PROGRAM P_Prog6
VAR

	fbKL6401 					: FB_LON_KL6401;

	fbREAD_159		: FB_READ_159_SNVT_pump_sensor;
	fbSEND_159		: FB_SEND_159_SNVT_pump_sensor;

	fbREAD_160		: FB_READ_160_SNVT_abs_humid;
	fbSEND_160		: FB_SEND_160_SNVT_abs_humid;

	fbREAD_161		: FB_READ_161_SNVT_flow_p;
	fbSEND_161		: FB_SEND_161_SNVT_flow_p;

	fbREAD_162		: FB_READ_162_SNVT_dev_c_mode;
	fbSEND_162		: FB_SEND_162_SNVT_dev_c_mode;

	fbREAD_163		: FB_READ_163_SNVT_valve_mode;
	fbSEND_163		: FB_SEND_163_SNVT_valve_mode;

	fbREAD_164		: FB_READ_164_SNVT_alarm_2;
	fbSEND_164		: FB_SEND_164_SNVT_alarm_2;

	fbREAD_165		: FB_READ_165_SNVT_state_64;
	fbSEND_165		: FB_SEND_165_SNVT_state_64;

	fbREAD_166		: FB_READ_166_SNVT_nv_type;
	fbSEND_166		: FB_SEND_166_SNVT_nv_type;
(*
	fbREAD_167		: FB_READ_109_SNVT_occupancy;
	fbSEND_167		: FB_SEND_109_SNVT_occupancy;
*)
	fbREAD_168		: FB_READ_168_SNVT_ent_opmode;
	fbSEND_168		: FB_SEND_168_SNVT_ent_opmode;

	fbREAD_169		: FB_READ_169_SNVT_ent_state;
	fbSEND_169		: FB_SEND_169_SNVT_ent_state;

	fbREAD_170		: FB_READ_170_SNVT_ent_status;
	fbSEND_170		: FB_SEND_170_SNVT_ent_status;

	fbREAD_171		: FB_READ_171_SNVT_flow_dir;
	fbSEND_171		: FB_SEND_171_SNVT_flow_dir;

	fbREAD_172		: FB_READ_172_SNVT_hvac_satsts;
	fbSEND_172		: FB_SEND_172_SNVT_hvac_satsts;

	fbREAD_173		: FB_READ_173_SNVT_dev_status;
	fbSEND_173		: FB_SEND_173_SNVT_dev_status;

	fbREAD_174		: FB_READ_174_SNVT_dev_fault;
	fbSEND_174		: FB_SEND_174_SNVT_dev_fault;

	fbREAD_175		: FB_READ_175_SNVT_dev_maint;
	fbSEND_175		: FB_SEND_175_SNVT_dev_maint;

	fbREAD_176		: FB_READ_176_SNVT_date_event;
	fbSEND_176		: FB_SEND_176_SNVT_date_event;

	fbREAD_177		: FB_READ_177_SNVT_sched_val;
	fbSEND_177		: FB_SEND_177_SNVT_sched_val;

(*
	fbREAD_178		: FB_READ_178;
	fbSEND_178		: FB_SEND_146_SNVT_elec_kwh_l;

	fbREAD_179		: FB_READ_147_SNVT_temp_diff_p;
	fbSEND_179		: FB_SEND_147_SNVT_temp_diff_p;
*)
	fbREAD_180		: FB_READ_180_SNVT_sblnd_state;
	fbSEND_180		: FB_SEND_180_SNVT_sblnd_state;

	fbREAD_181		: FB_READ_181_SNVT_rac_ctrl;
	fbSEND_181		: FB_SEND_181_SNVT_rac_ctrl;

	fbREAD_182		: FB_READ_182_SNVT_rac_req;
	fbSEND_182		: FB_SEND_182_SNVT_rac_req;

	fbREAD_183		: FB_READ_183_SNVT_count_32;
	fbSEND_183		: FB_SEND_183_SNVT_count_32;

	fbREAD_184		: FB_READ_184_SNVT_clothes_w_c;
	fbSEND_184		: FB_SEND_184_SNVT_clothes_w_c;

	fbREAD_185		: FB_READ_185_SNVT_clothes_w_m;
	fbSEND_185		: FB_SEND_185_SNVT_clothes_w_m;

	fbREAD_186		: FB_READ_186_SNVT_clothes_w_s;
	fbSEND_186		: FB_SEND_186_SNVT_clothes_w_s;

	fbREAD_187		: FB_READ_187_SNVT_clothes_w_a;
	fbSEND_187		: FB_SEND_187_SNVT_clothes_w_a;

	fbREAD_188		: FB_READ_188_SNVT_multiplier_s;
	fbSEND_188		: FB_SEND_188_SNVT_multiplier_s;

	fbREAD_189		: FB_READ_189_SNVT_switch_2;
	fbSEND_189		: FB_SEND_189_SNVT_switch_2;

	fbREAD_190		: FB_READ_190_SNVT_color_2;
	fbSEND_190		: FB_SEND_190_SNVT_color_2;

END_VAR

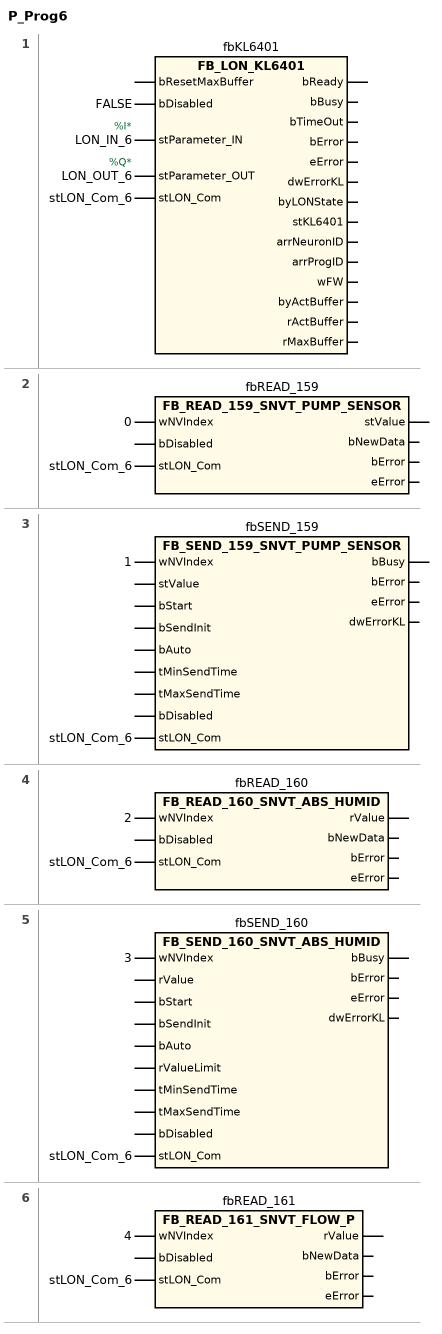
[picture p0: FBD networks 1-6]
// NETWORK 1
//   LON_IN_6: AT %I*
//   LON_OUT_6: AT %Q*
fbKL6401(
    bDisabled := FALSE,
    stParameter_IN := LON_IN_6,
    stParameter_OUT := LON_OUT_6,
    stLON_Com := stLON_Com_6); // FB_LON_KL6401

// NETWORK 2
fbREAD_159(wNVIndex := 0, stLON_Com := stLON_Com_6); // FB_READ_159_SNVT_PUMP_SENSOR

// NETWORK 3
fbSEND_159(wNVIndex := 1, stLON_Com := stLON_Com_6); // FB_SEND_159_SNVT_PUMP_SENSOR

// NETWORK 4
fbREAD_160(wNVIndex := 2, stLON_Com := stLON_Com_6); // FB_READ_160_SNVT_ABS_HUMID

// NETWORK 5
fbSEND_160(wNVIndex := 3, stLON_Com := stLON_Com_6); // FB_SEND_160_SNVT_ABS_HUMID

// NETWORK 6
fbREAD_161(wNVIndex := 4, stLON_Com := stLON_Com_6); // FB_READ_161_SNVT_FLOW_P

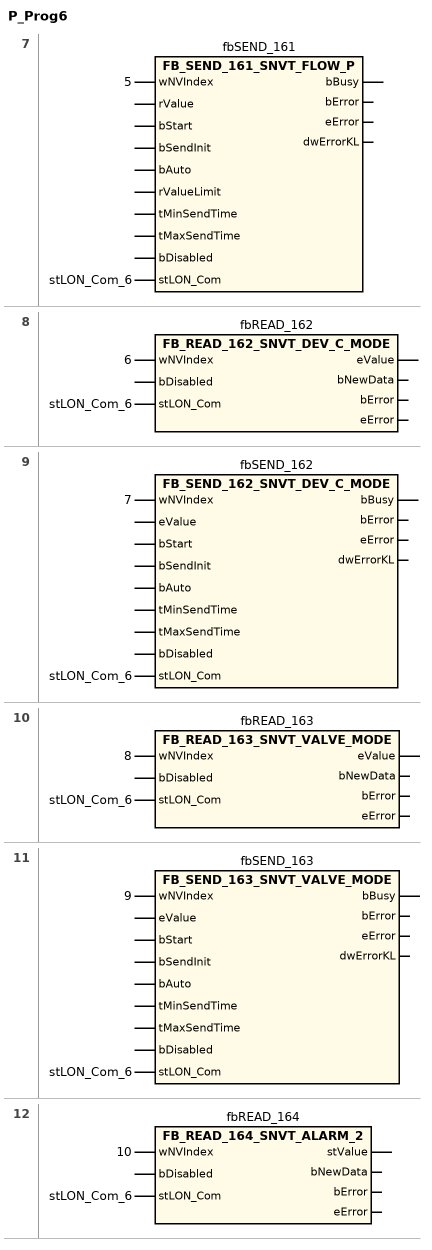
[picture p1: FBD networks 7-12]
// NETWORK 7
fbSEND_161(wNVIndex := 5, stLON_Com := stLON_Com_6); // FB_SEND_161_SNVT_FLOW_P

// NETWORK 8
fbREAD_162(wNVIndex := 6, stLON_Com := stLON_Com_6); // FB_READ_162_SNVT_DEV_C_MODE

// NETWORK 9
fbSEND_162(wNVIndex := 7, stLON_Com := stLON_Com_6); // FB_SEND_162_SNVT_DEV_C_MODE

// NETWORK 10
fbREAD_163(wNVIndex := 8, stLON_Com := stLON_Com_6); // FB_READ_163_SNVT_VALVE_MODE

// NETWORK 11
fbSEND_163(wNVIndex := 9, stLON_Com := stLON_Com_6); // FB_SEND_163_SNVT_VALVE_MODE

// NETWORK 12
fbREAD_164(wNVIndex := 10, stLON_Com := stLON_Com_6); // FB_READ_164_SNVT_ALARM_2

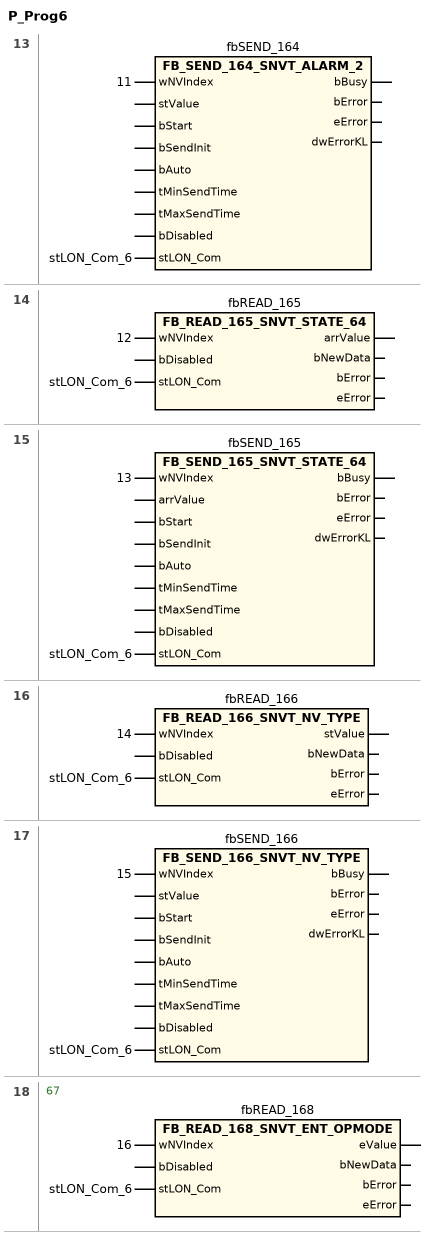
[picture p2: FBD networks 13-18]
// NETWORK 13
fbSEND_164(wNVIndex := 11, stLON_Com := stLON_Com_6); // FB_SEND_164_SNVT_ALARM_2

// NETWORK 14
fbREAD_165(wNVIndex := 12, stLON_Com := stLON_Com_6); // FB_READ_165_SNVT_STATE_64

// NETWORK 15
fbSEND_165(wNVIndex := 13, stLON_Com := stLON_Com_6); // FB_SEND_165_SNVT_STATE_64

// NETWORK 16
fbREAD_166(wNVIndex := 14, stLON_Com := stLON_Com_6); // FB_READ_166_SNVT_NV_TYPE

// NETWORK 17
fbSEND_166(wNVIndex := 15, stLON_Com := stLON_Com_6); // FB_SEND_166_SNVT_NV_TYPE

// NETWORK 18
// 					67
//
//
//   fbREAD_168: fbREAD_167 : FB_READ_109_SNVT_occupancy; fbSEND_167 : FB_SEND_109_SNVT_occupancy;
fbREAD_168(wNVIndex := 16, stLON_Com := stLON_Com_6); // FB_READ_168_SNVT_ENT_OPMODE

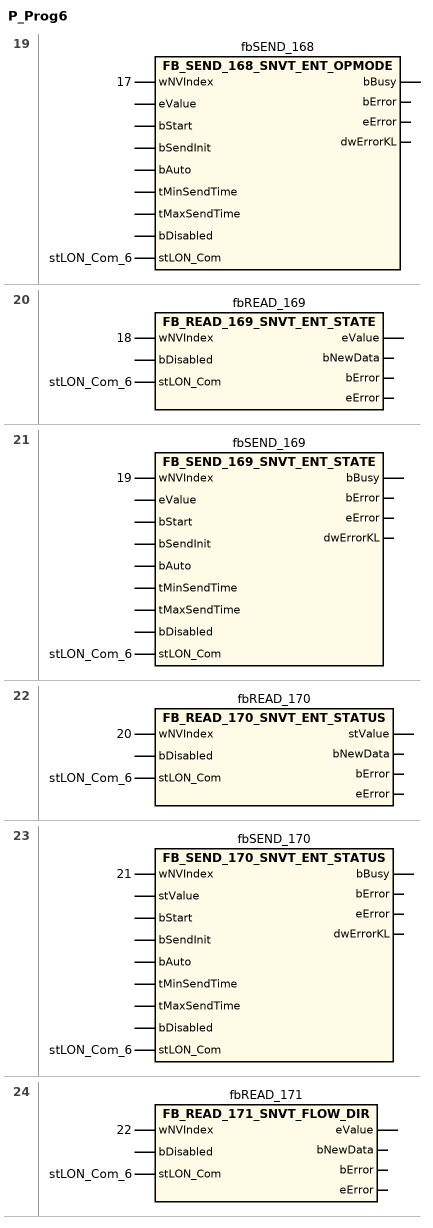
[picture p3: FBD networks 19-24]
// NETWORK 19
fbSEND_168(wNVIndex := 17, stLON_Com := stLON_Com_6); // FB_SEND_168_SNVT_ENT_OPMODE

// NETWORK 20
fbREAD_169(wNVIndex := 18, stLON_Com := stLON_Com_6); // FB_READ_169_SNVT_ENT_STATE

// NETWORK 21
fbSEND_169(wNVIndex := 19, stLON_Com := stLON_Com_6); // FB_SEND_169_SNVT_ENT_STATE

// NETWORK 22
fbREAD_170(wNVIndex := 20, stLON_Com := stLON_Com_6); // FB_READ_170_SNVT_ENT_STATUS

// NETWORK 23
fbSEND_170(wNVIndex := 21, stLON_Com := stLON_Com_6); // FB_SEND_170_SNVT_ENT_STATUS

// NETWORK 24
fbREAD_171(wNVIndex := 22, stLON_Com := stLON_Com_6); // FB_READ_171_SNVT_FLOW_DIR

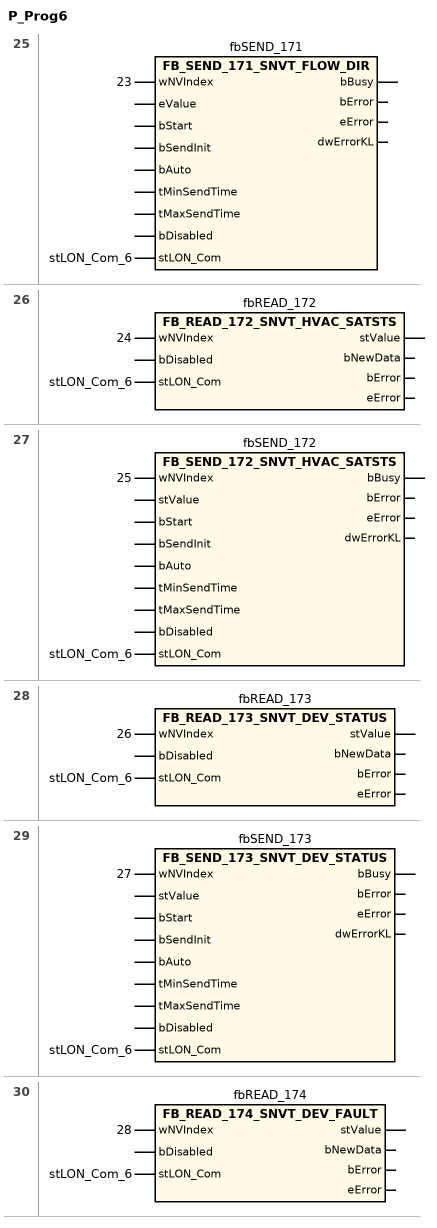
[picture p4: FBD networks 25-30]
// NETWORK 25
fbSEND_171(wNVIndex := 23, stLON_Com := stLON_Com_6); // FB_SEND_171_SNVT_FLOW_DIR

// NETWORK 26
fbREAD_172(wNVIndex := 24, stLON_Com := stLON_Com_6); // FB_READ_172_SNVT_HVAC_SATSTS

// NETWORK 27
fbSEND_172(wNVIndex := 25, stLON_Com := stLON_Com_6); // FB_SEND_172_SNVT_HVAC_SATSTS

// NETWORK 28
fbREAD_173(wNVIndex := 26, stLON_Com := stLON_Com_6); // FB_READ_173_SNVT_DEV_STATUS

// NETWORK 29
fbSEND_173(wNVIndex := 27, stLON_Com := stLON_Com_6); // FB_SEND_173_SNVT_DEV_STATUS

// NETWORK 30
fbREAD_174(wNVIndex := 28, stLON_Com := stLON_Com_6); // FB_READ_174_SNVT_DEV_FAULT

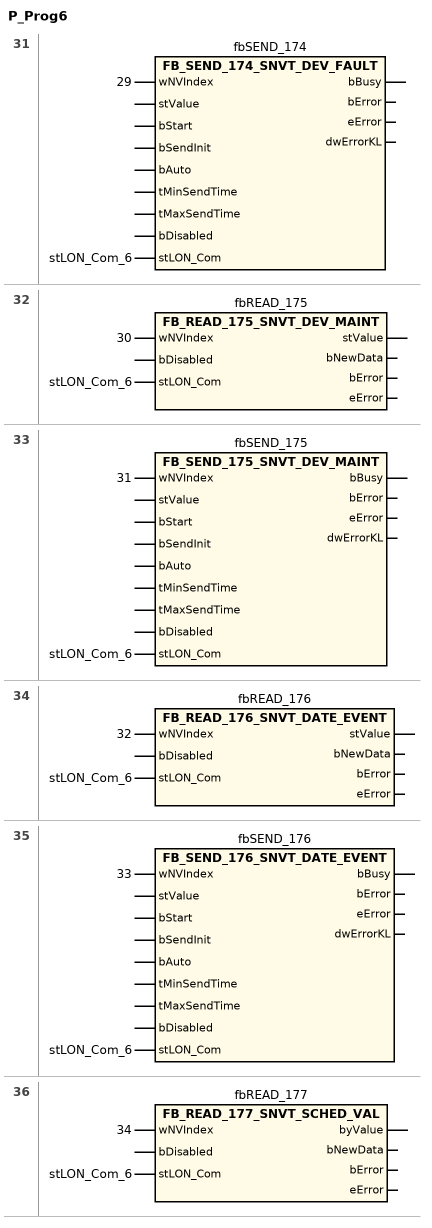
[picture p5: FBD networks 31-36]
// NETWORK 31
fbSEND_174(wNVIndex := 29, stLON_Com := stLON_Com_6); // FB_SEND_174_SNVT_DEV_FAULT

// NETWORK 32
fbREAD_175(wNVIndex := 30, stLON_Com := stLON_Com_6); // FB_READ_175_SNVT_DEV_MAINT

// NETWORK 33
fbSEND_175(wNVIndex := 31, stLON_Com := stLON_Com_6); // FB_SEND_175_SNVT_DEV_MAINT

// NETWORK 34
fbREAD_176(wNVIndex := 32, stLON_Com := stLON_Com_6); // FB_READ_176_SNVT_DATE_EVENT

// NETWORK 35
fbSEND_176(wNVIndex := 33, stLON_Com := stLON_Com_6); // FB_SEND_176_SNVT_DATE_EVENT

// NETWORK 36
fbREAD_177(wNVIndex := 34, stLON_Com := stLON_Com_6); // FB_READ_177_SNVT_SCHED_VAL

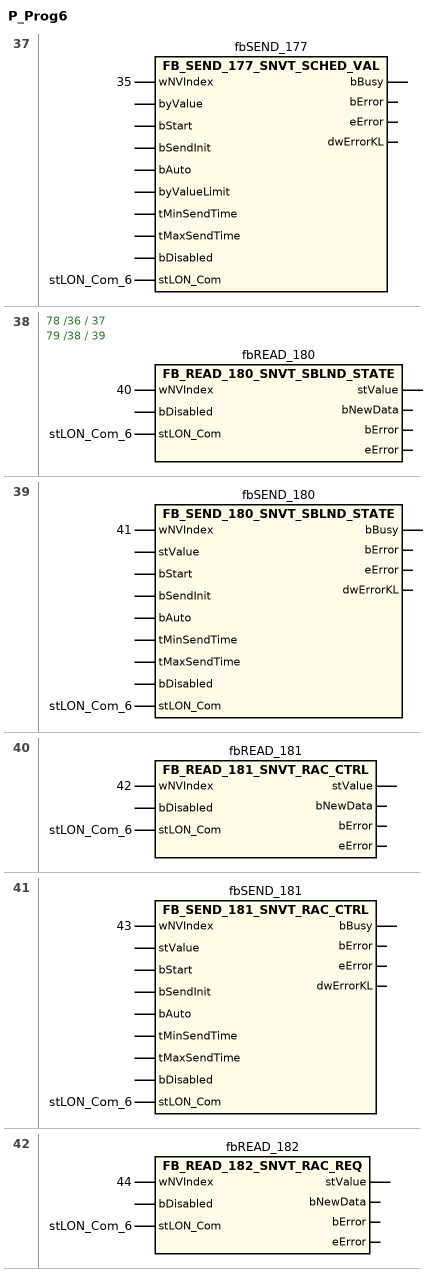
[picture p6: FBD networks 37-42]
// NETWORK 37
fbSEND_177(wNVIndex := 35, stLON_Com := stLON_Com_6); // FB_SEND_177_SNVT_SCHED_VAL

// NETWORK 38
// 					78 /36 / 37
// 79 /38 / 39
//
//
//   fbREAD_180: fbREAD_178 : FB_READ_178; fbSEND_178 : FB_SEND_146_SNVT_elec_kwh_l; fbREAD_179 : FB_READ_147_SNVT_temp_diff_p; fbSEND_179 : FB_SEND_147_SNVT_temp_diff_p;
fbREAD_180(wNVIndex := 40, stLON_Com := stLON_Com_6); // FB_READ_180_SNVT_SBLND_STATE

// NETWORK 39
fbSEND_180(wNVIndex := 41, stLON_Com := stLON_Com_6); // FB_SEND_180_SNVT_SBLND_STATE

// NETWORK 40
fbREAD_181(wNVIndex := 42, stLON_Com := stLON_Com_6); // FB_READ_181_SNVT_RAC_CTRL

// NETWORK 41
fbSEND_181(wNVIndex := 43, stLON_Com := stLON_Com_6); // FB_SEND_181_SNVT_RAC_CTRL

// NETWORK 42
fbREAD_182(wNVIndex := 44, stLON_Com := stLON_Com_6); // FB_READ_182_SNVT_RAC_REQ

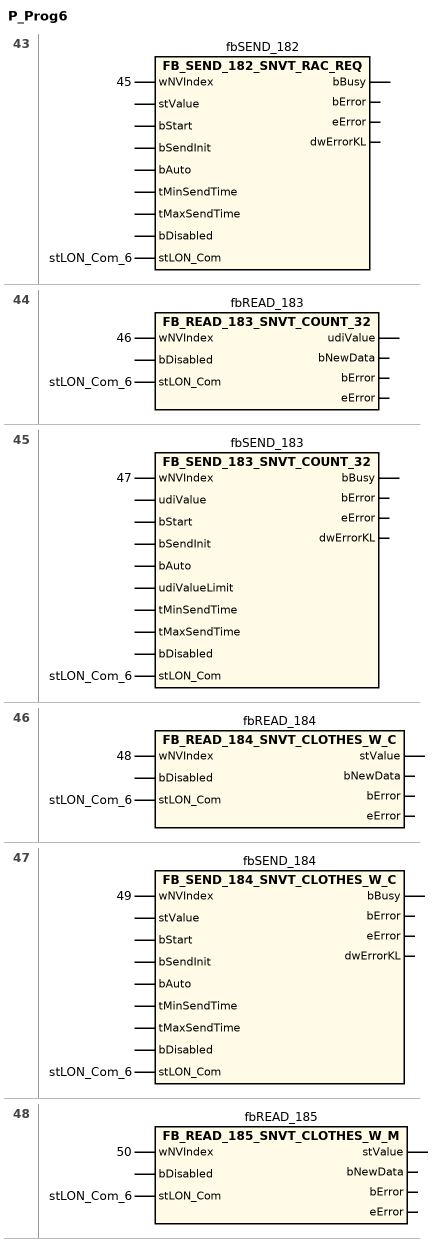
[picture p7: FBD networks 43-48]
// NETWORK 43
fbSEND_182(wNVIndex := 45, stLON_Com := stLON_Com_6); // FB_SEND_182_SNVT_RAC_REQ

// NETWORK 44
fbREAD_183(wNVIndex := 46, stLON_Com := stLON_Com_6); // FB_READ_183_SNVT_COUNT_32

// NETWORK 45
fbSEND_183(wNVIndex := 47, stLON_Com := stLON_Com_6); // FB_SEND_183_SNVT_COUNT_32

// NETWORK 46
fbREAD_184(wNVIndex := 48, stLON_Com := stLON_Com_6); // FB_READ_184_SNVT_CLOTHES_W_C

// NETWORK 47
fbSEND_184(wNVIndex := 49, stLON_Com := stLON_Com_6); // FB_SEND_184_SNVT_CLOTHES_W_C

// NETWORK 48
fbREAD_185(wNVIndex := 50, stLON_Com := stLON_Com_6); // FB_READ_185_SNVT_CLOTHES_W_M

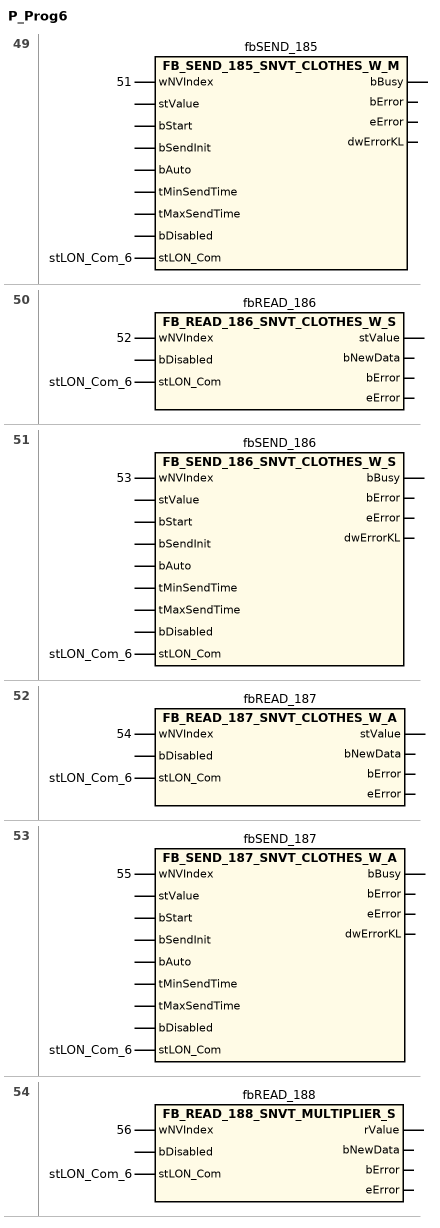
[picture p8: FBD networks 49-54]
// NETWORK 49
fbSEND_185(wNVIndex := 51, stLON_Com := stLON_Com_6); // FB_SEND_185_SNVT_CLOTHES_W_M

// NETWORK 50
fbREAD_186(wNVIndex := 52, stLON_Com := stLON_Com_6); // FB_READ_186_SNVT_CLOTHES_W_S

// NETWORK 51
fbSEND_186(wNVIndex := 53, stLON_Com := stLON_Com_6); // FB_SEND_186_SNVT_CLOTHES_W_S

// NETWORK 52
fbREAD_187(wNVIndex := 54, stLON_Com := stLON_Com_6); // FB_READ_187_SNVT_CLOTHES_W_A

// NETWORK 53
fbSEND_187(wNVIndex := 55, stLON_Com := stLON_Com_6); // FB_SEND_187_SNVT_CLOTHES_W_A

// NETWORK 54
fbREAD_188(wNVIndex := 56, stLON_Com := stLON_Com_6); // FB_READ_188_SNVT_MULTIPLIER_S

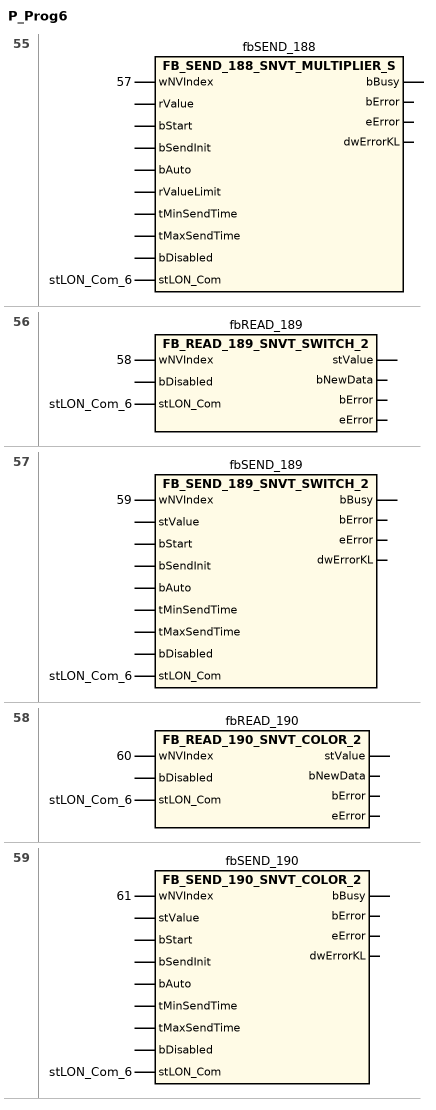
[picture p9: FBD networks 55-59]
// NETWORK 55
fbSEND_188(wNVIndex := 57, stLON_Com := stLON_Com_6); // FB_SEND_188_SNVT_MULTIPLIER_S

// NETWORK 56
fbREAD_189(wNVIndex := 58, stLON_Com := stLON_Com_6); // FB_READ_189_SNVT_SWITCH_2

// NETWORK 57
fbSEND_189(wNVIndex := 59, stLON_Com := stLON_Com_6); // FB_SEND_189_SNVT_SWITCH_2

// NETWORK 58
fbREAD_190(wNVIndex := 60, stLON_Com := stLON_Com_6); // FB_READ_190_SNVT_COLOR_2

// NETWORK 59
fbSEND_190(wNVIndex := 61, stLON_Com := stLON_Com_6); // FB_SEND_190_SNVT_COLOR_2

END_PROGRAM
